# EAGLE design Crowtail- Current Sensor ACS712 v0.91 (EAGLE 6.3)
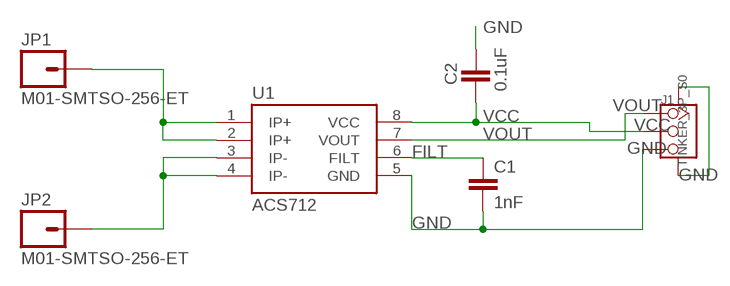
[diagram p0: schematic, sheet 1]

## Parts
C1  1nF  CAP0402-CAP  [0402-CAP]
C2  0.1uF  CAP0402-CAP  [0402-CAP]
J1  TINKER_3P_S0  [TINKER_3P_S0]
JP1  M01-SMTSO-256-ET  [SMTSO-256-ET]
JP2  M01-SMTSO-256-ET  [SMTSO-256-ET]
U1  ACS712  [SO08]

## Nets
FILT: C1.1 U1.6(FILT)
GND: C1.2 C2.2 J1.3 J1.SS1 J1.SS2 U1.5(GND)
N$1: JP1.P$1 U1.1(IP+) U1.2(IP+)
N$3: JP2.P$1 U1.3(IP-) U1.4(IP-)
VCC: C2.1 J1.2 U1.8(VCC)
VOUT: J1.1 U1.7(VOUT)

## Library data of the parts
C1 C2 = SparkFun:CAP: Capacitor
J1 = Connector:TINKER_3P_S0
JP1 JP2 = SparkFun:M01: Header 1
U1 = SparkFun:ACS712

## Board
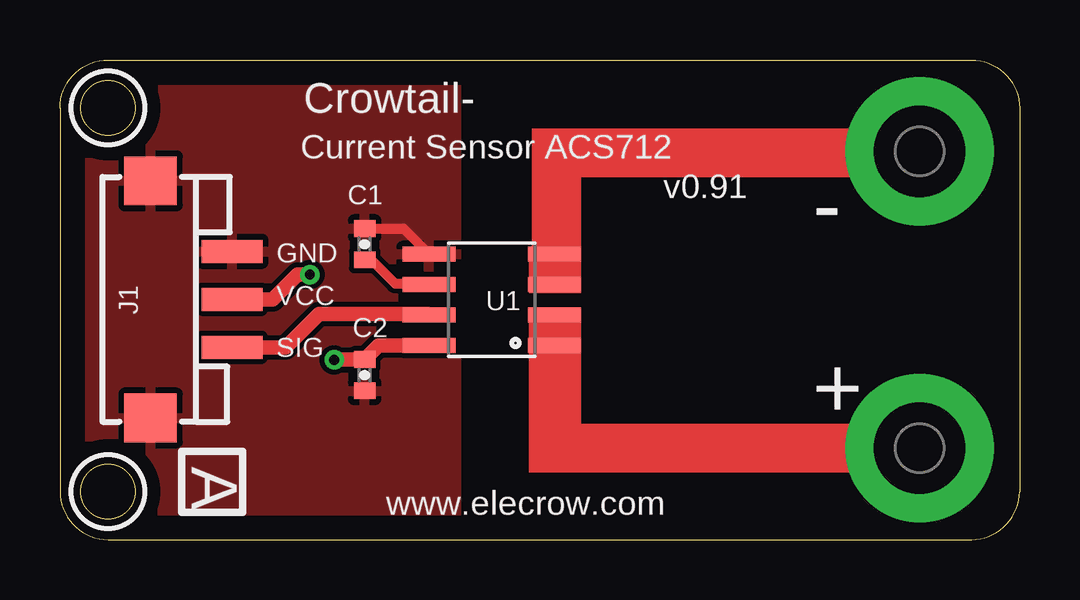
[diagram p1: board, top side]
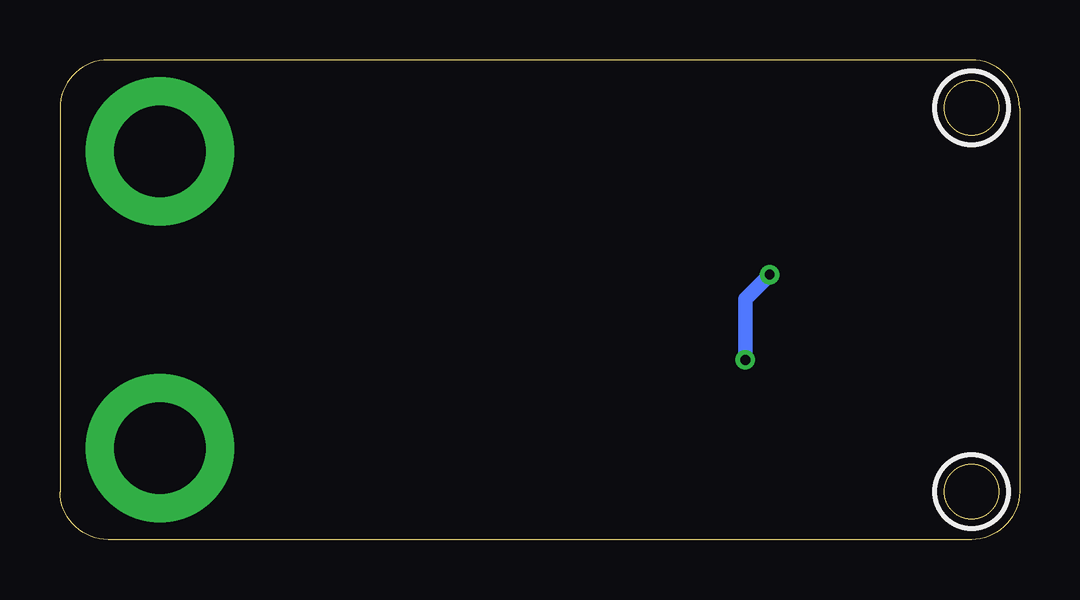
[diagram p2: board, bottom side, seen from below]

Size 40 x 20 mm. Coordinates in mm from the lower left corner, seen from the top.
Outline: 2,0 38,0 arc90 40,2 40,18 arc90 38,20 2,20 arc90 0,18 0,2 arc90 2,0
Outline: circle at 2,18 radius 1.14
Outline: circle at 2,2 radius 1.14
Copper layers (1*16): Top 0.035mm / dielectric 1.5mm / Bottom 0.035mm
Design rules "default *": minimum track width 10mil, minimum drill 24mil, track to track 8mil, track to pad 8mil, pad to pad 8mil, via to via 8mil, smd to smd 8mil, copper to edge 40mil, drill to drill 8mil, minimum pad ring 10mil, minimum via ring 8mil, stop-mask expansion 2mil, vias tented up to drill 100mil, thermal gap 10mil
tRestrict: area 0.5,16.5 to 3.5,19.5; area 0.5,0.5 to 3.5,3.5
bRestrict: area 0.5,16.5 to 3.5,19.5; area 0.5,0.5 to 3.5,3.5

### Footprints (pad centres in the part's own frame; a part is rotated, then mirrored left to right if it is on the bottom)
0402-CAP = smd 0.7 x 0.9: 1 -0.65,0; 2 0.65,0
TINKER_3P_S0 = smd 0.965 x 2.54: 1 -1.984,-3.175; 2 0.016,-3.175; 3 2.016,-3.175 | smd 2.032 x 2.184: SS1 -4.93,0.225; SS2 4.962,0.225
SMTSO-256-ET = drill 3.81 pad 6.198: P$1 0,0
SO08 = smd 0.61 x 2.21: 1 -1.905,-2.616; 2 -0.635,-2.616; 3 0.635,-2.616; 4 1.905,-2.616; 5 1.905,2.616; 6 0.635,2.616; 7 -0.635,2.616; 8 -1.905,2.616

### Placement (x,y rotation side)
C1  12.7,12.32 90 top
C2  12.7,6.86 270 top
J1  4,10 90 top
JP1  35.83,3.81 0 top
JP2  35.83,16.19 0 top
U1  18,10 90 top

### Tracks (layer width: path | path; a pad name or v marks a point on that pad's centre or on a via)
FILT
  Top 0.406: C1.1 12.97,11.67 13.97,10.67 15.35,10.67 U1.6
GND
  Top 0.406: C1.2 14.32,12.97 U1.5
  pour Top: 0,20.32 16.51,20.32 16.51,0 0,0
N$1
  Top 0.406: U1.2 U1.1 20.62,3.81 JP1.P$1
N$3
  Top 0.406: U1.4 U1.3 20.62,16.13 JP2.P$1
VCC  (via drill 0.41)
  Top 0.61: U1.8 13.29,8.1 C2.1 | J1.2 8.87,10.02 9.91,11.05 v10.41,11.05 | 12.69,7.49 C2.1 | v11.43,7.49 11.45,7.51 C2.1
  Bottom 0.61: v10.41,11.05 11.43,10.03 v11.43,7.49
VOUT
  Top 0.61: U1.7 15.35,9.4 10.79,9.4 9.4,8 7.19,8 J1.1
(copper drawn outside any net)
  shapes: Top area x5

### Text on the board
tPlace: Crowtail- | Current Sensor ACS712 | v0.91 | - | GND | VCC | SIG | + | A | www.elecrow.com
